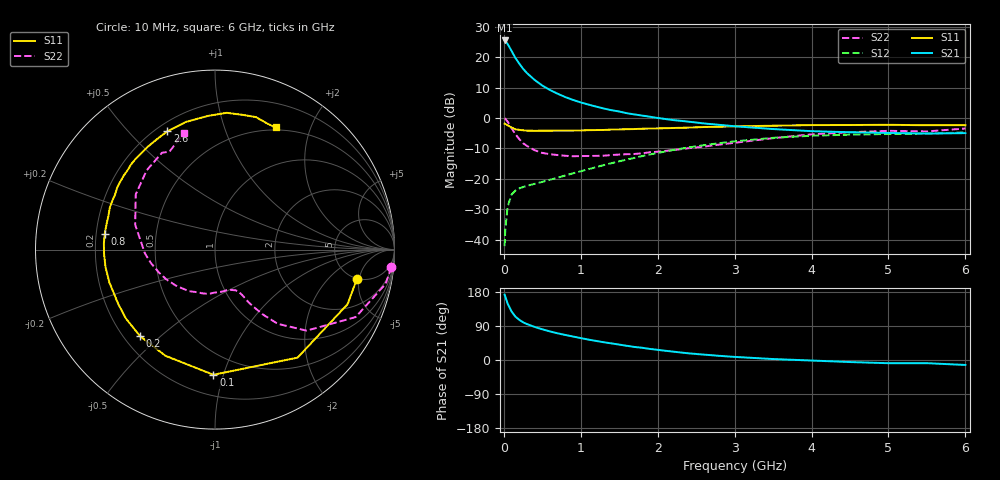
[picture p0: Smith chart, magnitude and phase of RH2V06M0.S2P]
! SIEMENS Small Signal Semiconductors
! BFR106
! Si NPN RF Bipolar Junction Transistor in SOT23
! VCE = 2 V  IC = 6 mA
! Common Emitter S-Parameters:  August  1996
# GHz  S  MA  R  50
!  f  S11  S21  S12  S22
! GHz  MAG  ANG  MAG  ANG  MAG  ANG  MAG  ANG
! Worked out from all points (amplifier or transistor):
!   36 points, 10 MHz to 6 GHz, reference 50 ohm
!   highest |S21| = 25.5 dB at 10 MHz (marker M1)
!   |S21| within 3 dB of that: start of sweep to 90.49 MHz
!   unconditionally stable (mu >= 1): 578.1 MHz to 2.277 GHz; 4.311 GHz to end of sweep
!   at 250 MHz: K = 0.56, MSG = 19.5 dB, |S12| = -22.7 dB
!   at 1.4 GHz: K = 1.15, MAG = 6.4 dB, |S12| = -14.9 dB
!   at 6 GHz: K = 1.02, MAG = -1.1 dB, |S12| = -4.8 dB
!   S11 on the Smith chart (normalised r, x): 10 MHz: 4.97, -4.64; 100 MHz: 0.34, -0.93; 200 MHz: 0.26, -0.43; 800 MHz: 0.24, +0.07; 2.6 GHz: 0.24, +0.65; 6 GHz: 0.47, +1.51
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0.01  0.8077 -11.6  18.84 172.4  0.0078 86.0  0.9872 -5.6
0.02  0.7988 -22.4  18.42 166.6  0.0154 79.0  0.9701 -11.3
0.05  0.7575 -52.6  16.41 148.5  0.035 64.5  0.8695 -25.6
0.1  0.6975 -90.7  12.71 128.1  0.0549 49.8  0.6815 -41.5
0.15  0.6529 -115.0  9.741 114.5  0.0641 42.1  0.5413 -49.8
0.2  0.6379 -130.9  7.858 106.1  0.0695 39.0  0.4509 -53.5
0.25  0.6275 -142.2  6.46 99.5  0.0731 37.5  0.3855 -56.0
0.3  0.6188 -150.3  5.483 94.8  0.0766 38.0  0.3479 -57.5
0.4  0.6164 -162.8  4.227 87.3  0.0826 39.7  0.2951 -59.1
0.5  0.6178 -170.9  3.416 81.0  0.089 42.4  0.2666 -60.8
0.6  0.6186 -177.8  2.886 75.4  0.0965 45.1  0.2539 -63.3
0.8  0.6206 171.7  2.205 66.0  0.1135 49.7  0.239 -69.8
1.1  0.6313 158.1  1.661 53.8  0.144 54.6  0.2374 -82.2
1.3  0.6354 151.3  1.431 46.8  0.168 56.1  0.2402 -91.3
1.6  0.6544 141.1  1.198 37.4  0.2075 56.3  0.2539 -106.4
2.2  0.6846 123.2  0.925 22.0  0.2972 51.5  0.2965 -137.4
2.6  0.7108 111.9  0.814 14.2  0.3568 45.7  0.3381 -158.0
3.5  0.746 93.0  0.658 2.5  0.4718 29.8  0.4659 162.7
4.5  0.7664 78.2  0.583 -5.4  0.5321 12.2  0.5833 130.7
5  0.7726 72.8  0.568 -8.5  0.5453 5.1  0.6151 118.7
5.5  0.7601 67.3  0.555 -8.4  0.5544 1.6  0.6019 114.9
6  0.7597 63.6  0.564 -13.1  0.5787 -5.7  0.6714 105.1
